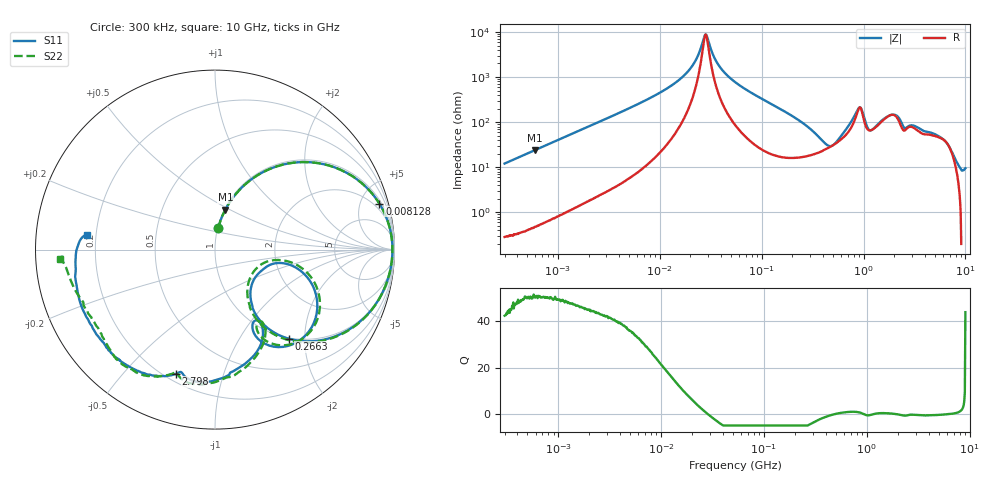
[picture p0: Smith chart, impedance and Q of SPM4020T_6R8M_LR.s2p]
! S-Parameter Data Generated by TDK Corporation
! Copyright(C) 2019 TDK Corporation.
! All Rights Reserved.
! TDK P/N: SPM4020T-6R8M-LR (Inductor)
! Property: L=6.8uH at 100kHz
! Size(LxWxT): 4.4x4.1x2mm
! Model Type: s2p (Touchstone File Format Version 1.0)
! Frequency: DC=Yes Start=0.3MHz Stop=10000MHz 802points Log-sweep
! Model Generated on Sep. 23, 2019
! Port Assignments:
!  1 ---@@@--- 2
! Applicable Conditions:
!  Temperature = 25 degC
!  DC Bias Current = 0 A
!  Small Signal Operation
! Terms and conditions regarding TDK Simulation Models
! (1)This simulation model is being provided solely for informational purposes. Please refer to the specifications of the products in terms of detailed characteristics of such products.
! (2)In no event shall TDK Corporation of any of its subsidiaries be liable for any loss or damage arising, directly or indirectly,
!  From any information contained in this simulation model, including, but not limited to loss or damages arising from any inaccuracies, omissions or errors in connection with such information.
! (3)Any and all copyrights on this simulation model are owned by TDK Corporation.
!  Duplication or redistribution of this simulation model without prior written permission from TDK Corporation is prohibited.
! (4)This simulation model is subject to any modification or change without any prior notice.
! (5)Neither TDK Corporation nor any of its subsidiaries shall make any warranty, express or implied,
!  Including but not limited to the correctness, implied warranties of merchantability and fitness for a particular purpose with respect to this simulation models.
! (6)The use of this simulation model shall be deemed to have consented to the terms and conditions hereof.
# Hz S MA R 50
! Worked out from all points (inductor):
!   801 points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, 300 kHz to 10 GHz, reference 50 ohm
!   read as one part in series: L = 6.4 uH near 318.3 kHz
!   highest Q = 50.7 at 592.8 kHz (marker M1), where L = 6.39 uH
!   self-resonance near 28.2 MHz
!   S11 on the Smith chart (normalised r, x): 300 kHz: 1.01, +0.24; 8.128 MHz: 1.31, +7.06; 266.3 MHz: 0.98, -1.68; 2.798 GHz: 0.24, -0.70; 10 GHz: 0.17, +0.05
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300000  0.1191 81.8  0.9901 -6.9  0.99 -6.9  0.1189 81.8
592755  0.2303 75.5  0.9686 -13.4  0.9684 -13.4  0.2301 75.5
1713600  0.5589 54.7  0.8171 -34.0  0.8171 -34.0  0.5589 54.7
8128066  0.9513 15.6  0.2741 -72.2  0.2742 -72.2  0.9513 15.6
9671944  0.9643 12.6  0.2248 -74.8  0.2249 -74.8  0.9643 12.6
1.945436e7  0.9873 3.2  0.06878 -78.2  0.06879 -78.2  0.9873 3.1
2.78833e7  0.9887 -0.9  0.01146 -13.1  0.01146 -13.0  0.9887 -1.0
3.904515e7  0.9859 -4.8  0.05951 73.1  0.05952 73.1  0.9859 -4.9
5.477226e7  0.978 -9.3  0.1257 74.2  0.1257 74.2  0.978 -9.4
1.275226e8  0.9047 -26.0  0.3628 59.5  0.3628 59.5  0.9044 -26.3
2.663116e8  0.6451 -50.4  0.6589 28.9  0.6588 28.9  0.6423 -51.4
3.126428e8  0.5476 -55.3  0.7128 19.7  0.7128 19.7  0.543 -56.6
5.165633e8  0.2731 -36.6  0.7438 -14.6  0.7438 -14.6  0.2486 -36.0
6.738867e8  0.3772 -11.4  0.6294 -34.5  0.6294 -34.5  0.3769 -9.0
8.872678e8  0.6685 -32.0  0.3229 -41.5  0.3229 -41.5  0.6685 -29.1
1.001841e9  0.6614 -55.0  0.3778 -12.2  0.3778 -12.2  0.6728 -51.8
1.133369e9  0.4971 -64.8  0.5282 -25.2  0.5283 -25.2  0.5139 -62.5
1.35547e9  0.4748 -58.3  0.4779 -46.8  0.4779 -46.9  0.4887 -56.9
1.767019e9  0.6405 -72.0  0.3224 -57.0  0.3225 -57.0  0.6496 -71.0
2.798208e9  0.7268 -107.6  0.3032 -61.3  0.3033 -61.3  0.7343 -109.3
6.091595e9  0.8105 -141.3  0.2262 -91.0  0.2264 -91.1  0.7935 -142.4
1e10  0.7165 173.7  0.1385 -128.4  0.1385 -128.6  0.8649 -176.7
